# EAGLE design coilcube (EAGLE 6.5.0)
REV: 2v0; TITLE: Coilcube

## Sheet 1 of 2: EPIC & Programmer
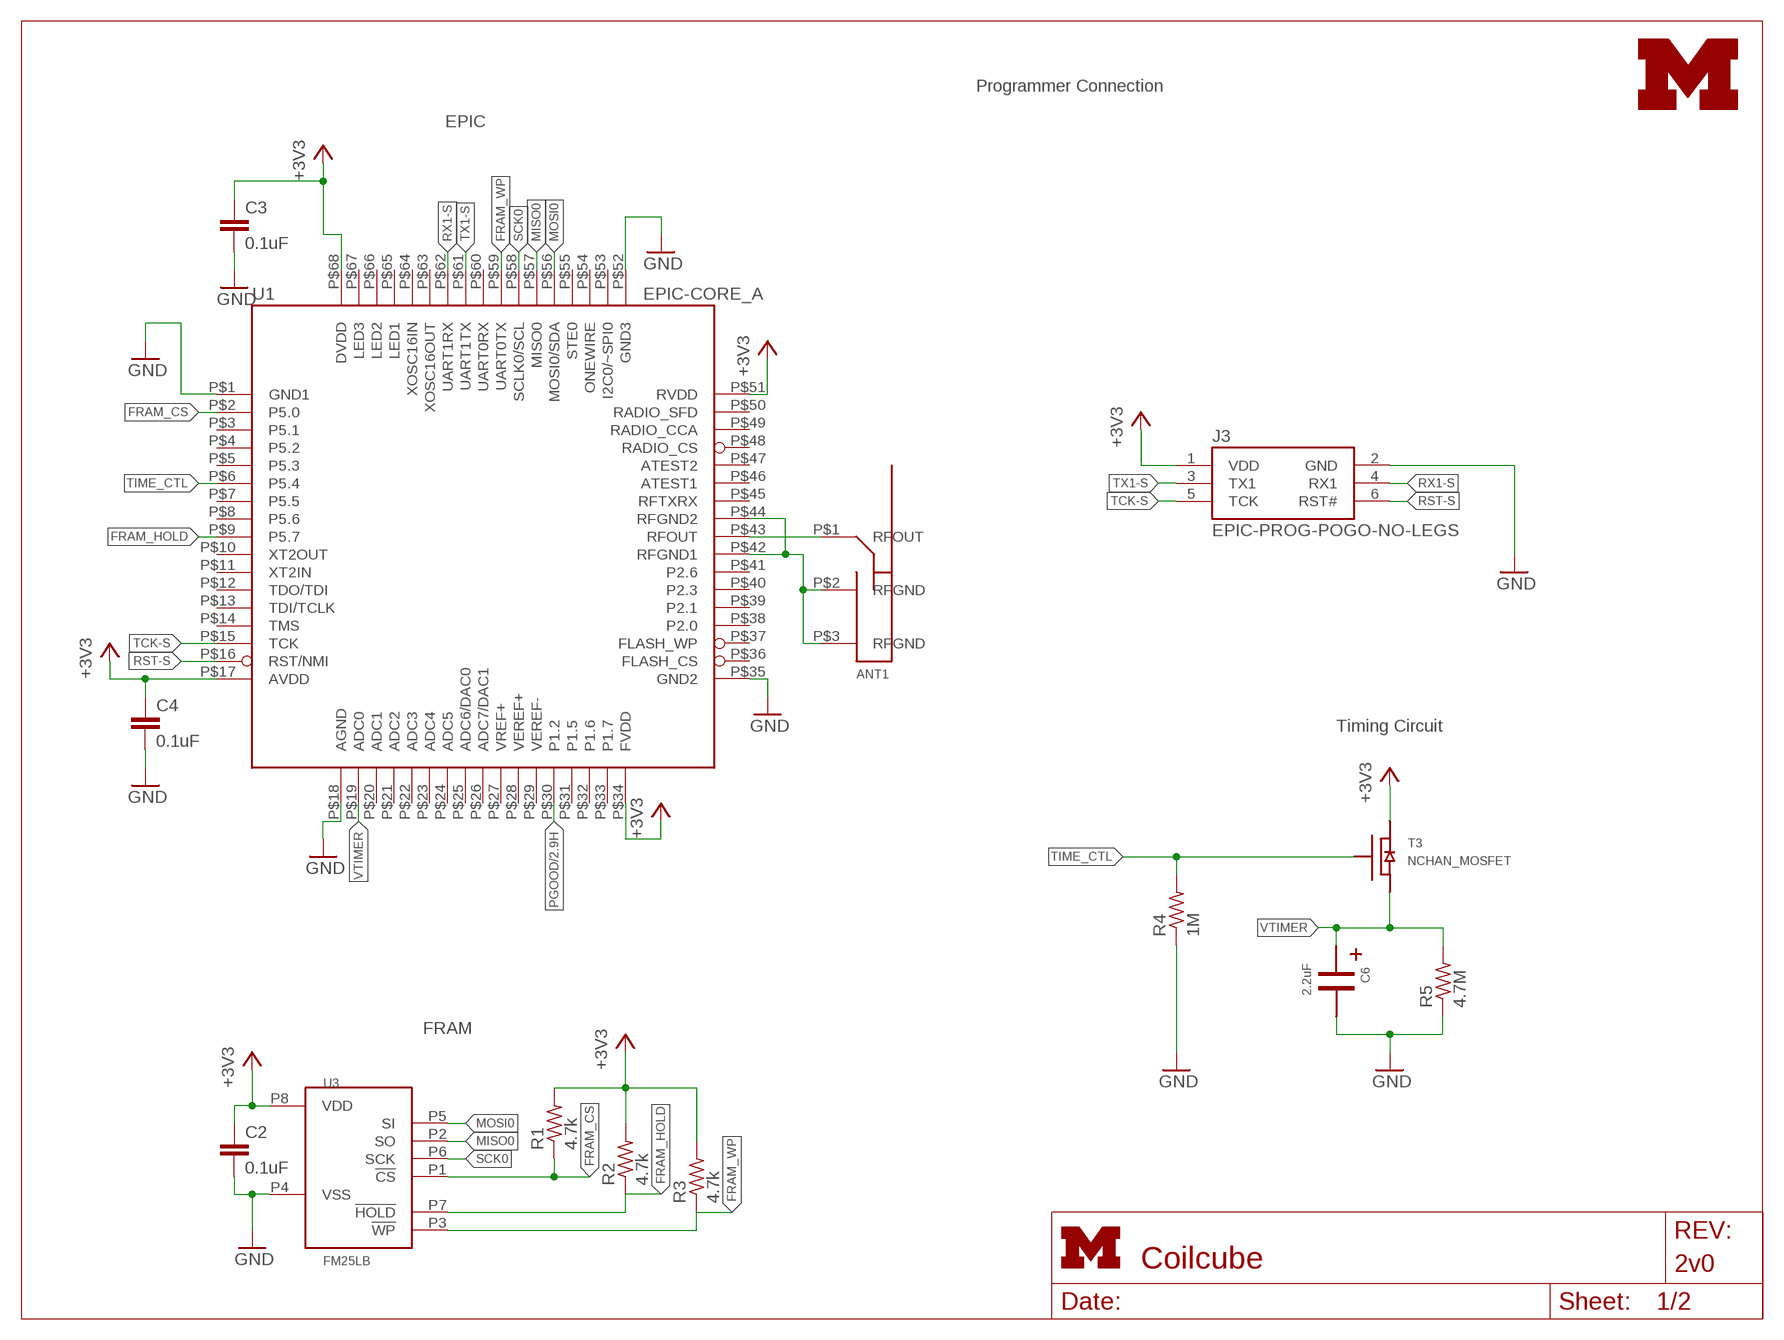
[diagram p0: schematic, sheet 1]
FRAME1 (LETTER_L): HEIGHT: 8.5in; WIDTH: 11in

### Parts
ANT1  PIFA-2.4GHZ  [PIFA-2.4GHZ]
C2  0.1uF  C-EUC0603  [C0603]
C3  0.1uF  C-EUC0603  [C0603]
C4  0.1uF  C-EUC0603  [C0603]
C6  2.2uF  CAP_POLEA1MM5  [CPOL_EEA_1MM5]
J3  EPIC-PROG-POGO-NO-LEGS  [TC2030-IDC-NL]
R1  4.7k  R-US_R0603  [R0603]
R2  4.7k  R-US_R0603  [R0603]
R3  4.7k  R-US_R0603  [R0603]
R4  1M  R-US_R0603  [R0603]
R5  4.7M  R-US_R0603  [R0603]
T3  NCHAN_MOSFET  [NCHAN_MOSFET]
U1  EPIC-CORE_A  [EPIC-LCC68]
U3  FM25LB  [SOIC_8]
U$1  UMICH_SOLID_MEDIUM  [UMICH_SOLID_200MIL]

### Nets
+3V3: C2.1 C3.1 C4.1 J3.1(VDD) R1.2 R2.2 R3.2 T3.D U1.P$17(AVDD) U1.P$34(FVDD) U1.P$51(RVDD) U1.P$68(DVDD) U3.P8(VDD) ; also sheet 2
FRAM_CS: R1.1 U1.P$2(P5.0) U3.P1(!CS)
FRAM_HOLD: R2.1 U1.P$9(P5.7) U3.P7(!HOLD)
FRAM_WP: R3.1 U1.P$59(UART0TX) U3.P3(!WP)
GND: C2.2 C3.2 C4.2 C6.- J3.2(GND) R4.1 R5.1 U1.P$1(GND1) U1.P$18(AGND) U1.P$35(GND2) U1.P$52(GND3) U3.P4(VSS) ; also sheet 2
MISO0: U1.P$57(MISO0) U3.P2(SO)
MOSI0: U1.P$56(MOSI0/SDA) U3.P5(SI)
N$1: ANT1.P$1(RFOUT) U1.P$43(RFOUT)
PGOOD: U1.P$30(P1.2) ; also sheet 2
RFGND: ANT1.P$2(RFGND) ANT1.P$3(RFGND) U1.P$42(RFGND1) U1.P$44(RFGND2)
RST-S: J3.6(RST#) U1.P$16(RST/NMI)
RX1-S: J3.4(RX1) U1.P$62(UART1RX)
SCK0: U1.P$58(SCLK0/SCL) U3.P6(SCK)
TCK-S: J3.5(TCK) U1.P$15(TCK)
TIME_CTL: R4.2 T3.G U1.P$6(P5.4)
TX1-S: J3.3(TX1) U1.P$61(UART1TX)
VTIMER: C6.+ R5.2 T3.S U1.P$19(ADC0)
Unconnected: U1.P$3(P5.1) U1.P$4(P5.2) U1.P$5(P5.3) U1.P$7(P5.5) U1.P$8(P5.6) U1.P$10(XT2OUT) U1.P$11(XT2IN) U1.P$12(TDO/TDI) U1.P$13(TDI/TCLK) U1.P$14(TMS) U1.P$20(ADC1) U1.P$21(ADC2) U1.P$22(ADC3) U1.P$23(ADC4) U1.P$24(ADC5) U1.P$25(ADC6/DAC0) U1.P$26(ADC7/DAC1) U1.P$27(VREF+) U1.P$28(VEREF+) U1.P$29(VEREF-) U1.P$31(P1.5) U1.P$32(P1.6) U1.P$33(P1.7) U1.P$36(FLASH_CS) U1.P$37(FLASH_WP) U1.P$38(P2.0) U1.P$39(P2.1) U1.P$40(P2.3) U1.P$41(P2.6) U1.P$45(RFTXRX) U1.P$46(ATEST1) U1.P$47(ATEST2) U1.P$48(RADIO_CS) U1.P$49(RADIO_CCA) U1.P$50(RADIO_SFD) U1.P$53(I2C0/~SPI0) U1.P$54(ONEWIRE) U1.P$55(STE0) U1.P$60(UART0RX) U1.P$63(XOSC16OUT) U1.P$64(XOSC16IN) U1.P$65(LED1) U1.P$66(LED2) U1.P$67(LED3)

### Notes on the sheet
- Programmer Connection
- EPIC
- Timing Circuit
- FRAM

## Sheet 2 of 2: Power Supply
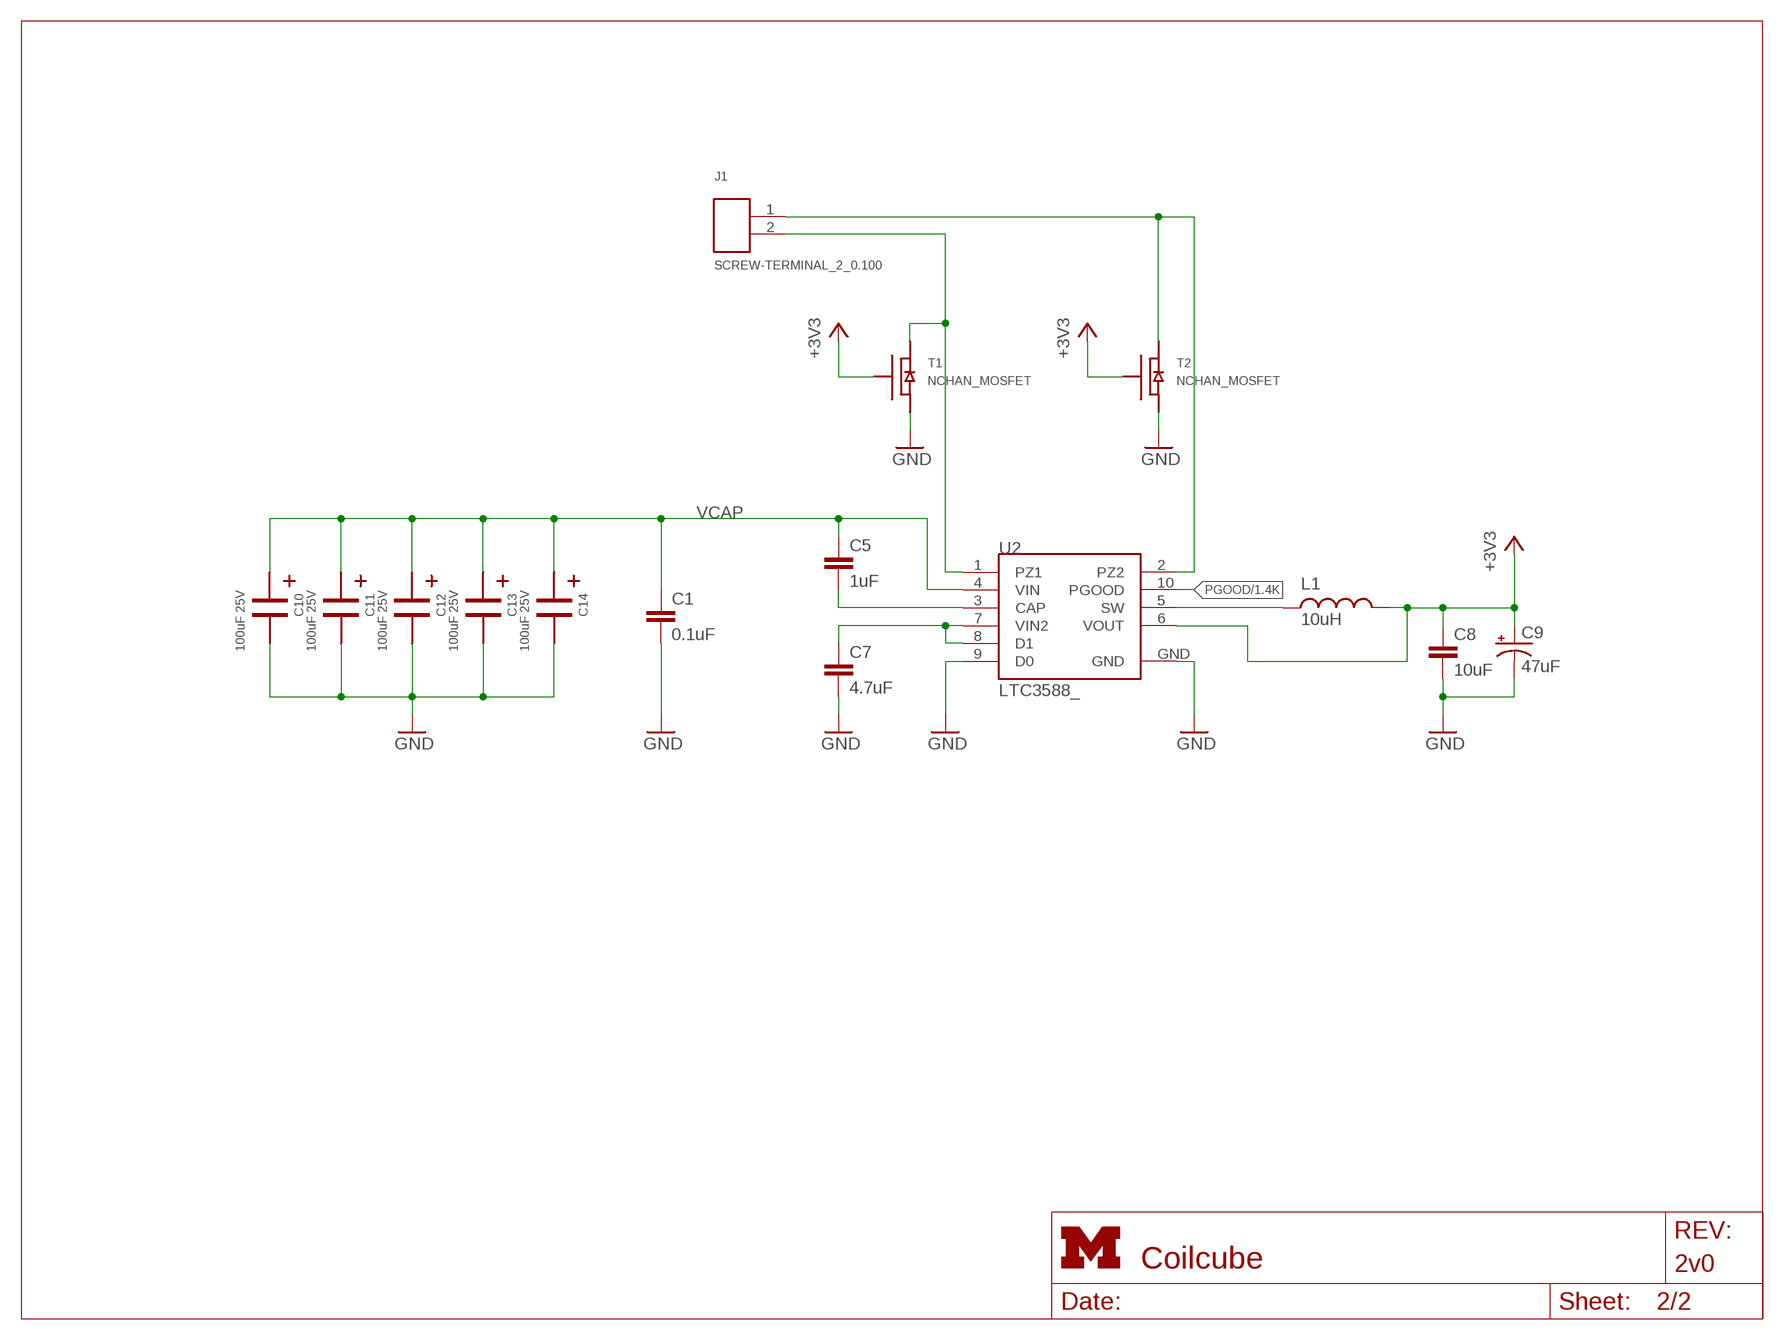
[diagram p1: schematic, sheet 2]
FRAME5 (LETTER_L): HEIGHT: 8.5in; WIDTH: 11in

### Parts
C1  0.1uF  C-EUC0603  [C0603]
C5  1uF  C-EUC0603  [C0603]
C7  4.7uF  C-EUC0603  [C0603]
C8  10uF  C-EUC1206  [C1206]
C9  47uF  CAP_POL1206  [EIA3216]
C10  100uF 25V  2917_CAP_POL  [2917_CAP_POL]
C11  100uF 25V  2917_CAP_POL  [2917_CAP_POL]
C12  100uF 25V  2917_CAP_POL  [2917_CAP_POL]
C13  100uF 25V  2917_CAP_POL  [2917_CAP_POL]
C14  100uF 25V  2917_CAP_POL  [2917_CAP_POL]
J1  SCREW-TERMINAL_2_0.100  [CONN_BLOCK_2]
L1  10uH  INDUCTOR1210  [1210]
T1  NCHAN_MOSFET  [NCHAN_MOSFET]
T2  NCHAN_MOSFET  [NCHAN_MOSFET]
U2  LTC3588_  [MSOP-10-GNDPAD]

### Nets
+3V3: C8.1 C9.A(+) L1.2 T1.G T2.G U2.6(VOUT) ; also sheet 1
GND: C1.2 C7.2 C8.2 C9.C(-) C10.- C11.- C12.- C13.- C14.- T1.S T2.S U2.9(D0) U2.GND ; also sheet 1
N$20: L1.1 U2.5(SW)
N$22: C5.2 U2.3(CAP)
PGOOD: U2.10(PGOOD) ; also sheet 1
PZ1: J1.2 T1.D U2.1(PZ1)
PZ2: J1.1 T2.D U2.2(PZ2)
VCAP: C1.1 C5.1 C10.+ C11.+ C12.+ C13.+ C14.+ U2.4(VIN)
VIN2: C7.1 U2.7(VIN2) U2.8(D1)

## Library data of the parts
ANT1 = berkeley-epic:PIFA-2.4GHZ
C1-C4 = rcl:C-EU: CAPACITOR, European symbol; DIGIKEY: 445-1316-1-ND
C5 = rcl:C-EU: CAPACITOR, European symbol; DIGIKEY: 445-1321-1-ND
C6 = coilcube:CAP_POL; DIGIKEY: P14506-ND
C7 = rcl:C-EU: CAPACITOR, European symbol; DIGIKEY: 445-5178-1-ND
C8 = rcl:C-EU: CAPACITOR, European symbol; DIGIKEY: 399-8152-1-ND
C9 = SparkFun-Passives:CAP_POL: Capacitor Polarized; DIGIKEY: 399-3700-1-ND
C10-C14 = coilcube:2917_CAP_POL; DIGIKEY: 399-5175-1-ND
J1 = headers:SCREW-TERMINAL_2_0.100: 2x 0.100 in screw terminal block; DIGIKEY: 277-1273-ND
J3 = epic:EPIC-PROG-POGO: Epic programmer based on the Tag Connect pogo pin cable.; TAG-CONNECT: TC2030-IDC-NL
L1 = SparkFun-Passives:INDUCTOR: Inductors; DIGIKEY: 587-1625-1-ND
R1-R5 = rcl:R-US_: RESISTOR, American symbol; DIGIKEY: P4.7KGCT-ND
T1 T2 = Power_Metering:NCHAN_MOSFET; DIGIKEY: SI1302DL-T1-GE3CT-ND
T3 = Power_Metering:NCHAN_MOSFET; DIGIKEY: 568-3244-1-ND
U1 = berkeley-epic:EPIC-CORE_A
U2 = SparkFun-PowerIC:LTC3588: Energy Harvesting Power Supply; DIGIKEY: LTC3588EMSE-1#PBF-ND
U3 = coilcube:FM25LB; DIGIKEY: 428-3210-ND
U$1 = logos:UMICH_SOLID

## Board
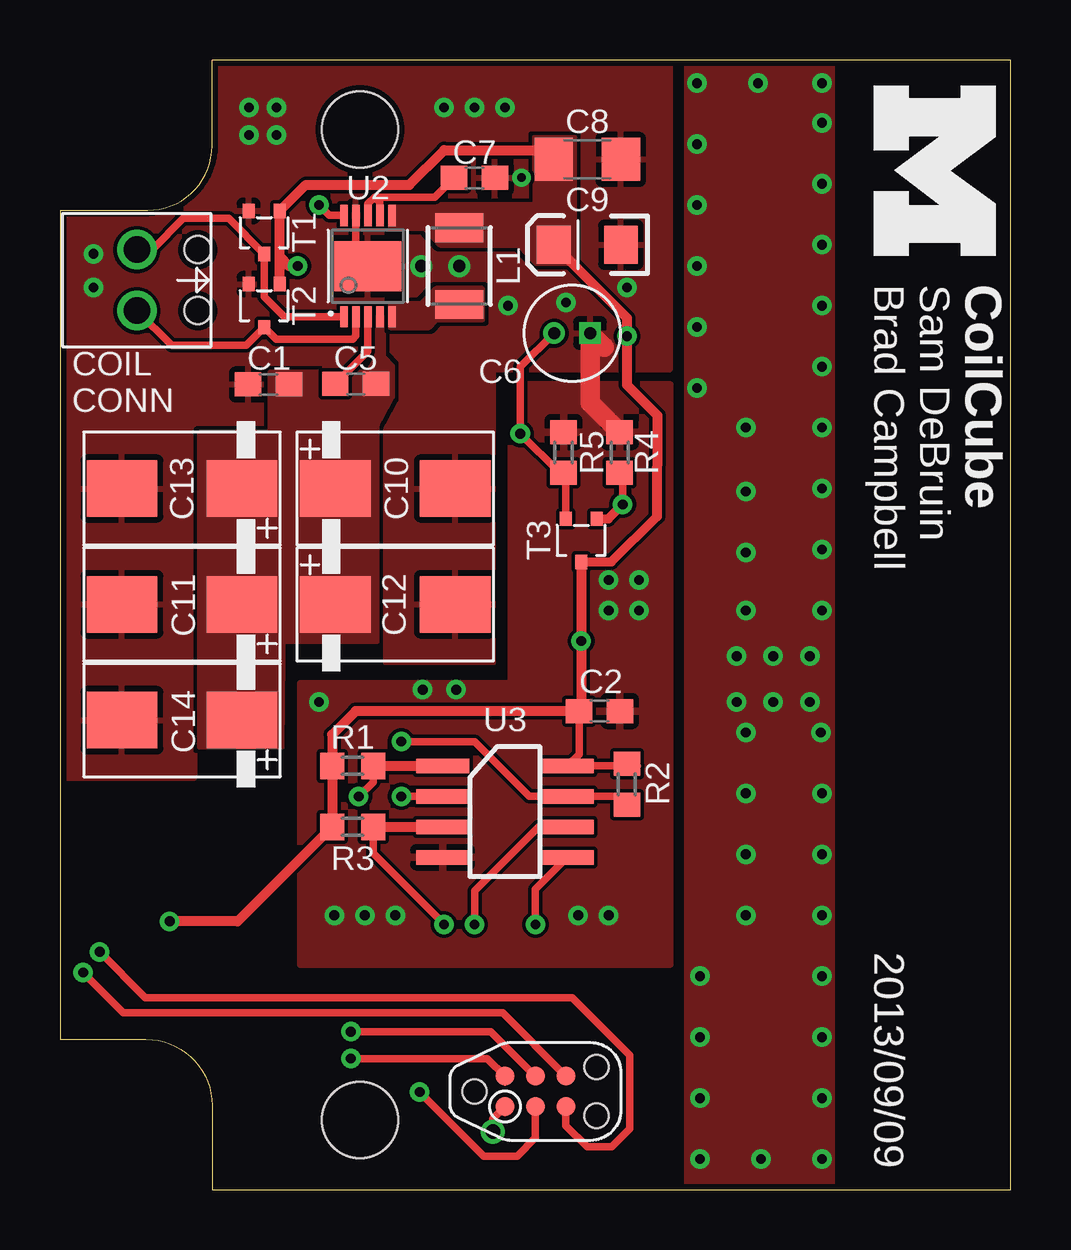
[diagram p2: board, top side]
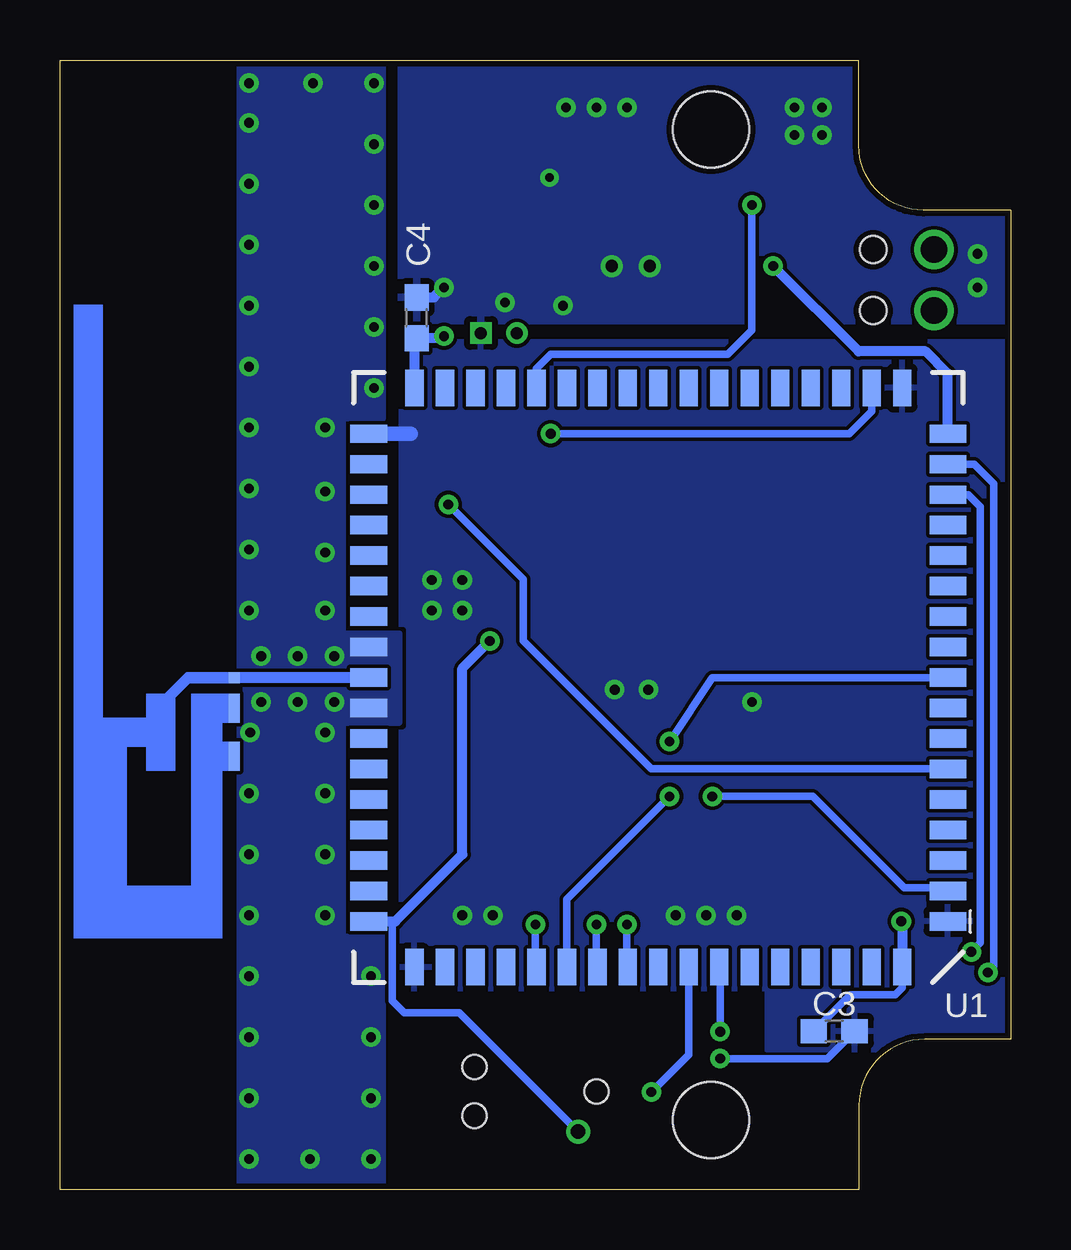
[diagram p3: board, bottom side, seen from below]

Size 39.62 x 47.07 mm. Coordinates in mm from the lower left corner, seen from the top.
Outline: 6.34,0 39.62,0 39.62,47.07 6.34,47.07 6.34,43.49 arc-90 3.65,40.8 0,40.8 0,6.26 3.58,6.26 arc-90 6.34,3.51 6.34,0
Copper layers (1*16): Top 0.0178mm / dielectric 59mil / Bottom 0.0178mm
Design rules "sunstone-2lyr_v1.0.0.3 *": minimum track width 6mil, minimum drill 14mil, track to track 6mil, track to pad 6mil, pad to pad 6mil, via to via 6mil, smd to smd 6mil, copper to edge 10mil, drill to drill 16mil, minimum pad ring 8mil, minimum via ring 8mil, stop-mask expansion 3mil, vias tented up to drill 20mil, thermal gap 10mil
Holes 3.17 mm at 12.5,44.17 12.5,2.9
tKeepout: area 10.1,0.5 to 14.9,5.3; area 10.1,41.8 to 14.9,46.6
Milling: 12 lines

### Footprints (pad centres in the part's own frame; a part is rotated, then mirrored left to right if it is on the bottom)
PIFA-2.4GHZ = smd 0.46 x 0.46: P$1 -2.65,-1.495 | smd 0.46 x 1.2: P$2 -2.655,1.785; P$3 -2.65,-0.215
C0603 = smd 1.1 x 1: 1 -0.85,0; 2 0.85,0
CPOL_EEA_1MM5 = drill 0.5: + 0.75,0 | drill 0.5 square: - -0.75,0
C1206 = smd 1.6 x 1.8: 1 -1.4,0; 2 1.4,0
EIA3216 = smd 1.4 x 1.6: A 1.4,0; C -1.4,0
2917_CAP_POL = smd 2.95 x 2.35: + -2.5,0; - 2.5,0
CONN_BLOCK_2 = drill 1.1: 1 -1.27,0; 2 1.27,0 | hole 1.12: -1.27,-2.54; 1.27,-2.54
TC2030-IDC-NL = smd 0.787 x 0.787: 1 -1.27,-0.635; 2 -1.27,0.635; 3 0,-0.635; 4 0,0.635; 5 1.27,-0.635; 6 1.27,0.635 | hole 1.016: -2.54,0; 2.54,1.016; 2.54,-1.016
1210 = smd 1.2 x 2: 1 -1.6,0; 2 1.6,0
R0603 = smd 1 x 1.1: 1 -0.85,0; 2 0.85,0
NCHAN_MOSFET = smd 0.6 x 0.5: D -0.9,0; G 0.9,-0.65; S 0.9,0.65
EPIC-LCC68 = smd 1.524 x 0.762: P$1 -12.065,10.16; P$2 -12.065,8.89; P$3 -12.065,7.62; P$4 -12.065,6.35; P$5 -12.065,5.08; P$6 -12.065,3.81; P$7 -12.065,2.54; P$8 -12.065,1.27; P$9 -12.065,0; P$10 -12.065,-1.27; P$11 -12.065,-2.54; P$12 -12.065,-3.81; P$13 -12.065,-5.08; P$14 -12.065,-6.35; P$15 -12.065,-7.62; P$16 -12.065,-8.89; P$17 -12.065,-10.16; P$35 12.065,-10.16; P$36 12.065,-8.89; P$37 12.065,-7.62; P$38 12.065,-6.35; P$39 12.065,-5.08; P$40 12.065,-3.81; P$41 12.065,-2.54; P$42 12.065,-1.27; P$43 12.065,0; P$44 12.065,1.27; P$45 12.065,2.54; P$46 12.065,3.81; P$47 12.065,5.08; P$48 12.065,6.35; P$49 12.065,7.62; P$50 12.065,8.89; P$51 12.065,10.16 | smd 0.762 x 1.524: P$18 -10.16,-12.065; P$19 -8.89,-12.065; P$20 -7.62,-12.065; P$21 -6.35,-12.065; P$22 -5.08,-12.065; P$23 -3.81,-12.065; P$24 -2.54,-12.065; P$25 -1.27,-12.065; P$26 0,-12.065; P$27 1.27,-12.065; P$28 2.54,-12.065; P$29 3.81,-12.065; P$30 5.08,-12.065; P$31 6.35,-12.065; P$32 7.62,-12.065; P$33 8.89,-12.065; P$34 10.16,-12.065; P$52 10.16,12.065; P$53 8.89,12.065; P$54 7.62,12.065; P$55 6.35,12.065; P$56 5.08,12.065; P$57 3.81,12.065; P$58 2.54,12.065; P$59 1.27,12.065; P$60 0,12.065; P$61 -1.27,12.065; P$62 -2.54,12.065; P$63 -3.81,12.065; P$64 -5.08,12.065; P$65 -6.35,12.065; P$66 -7.62,12.065; P$67 -8.89,12.065; P$68 -10.16,12.065
MSOP-10-GNDPAD = smd 0.305 x 0.889: 1 -1,-2.11; 2 -0.5,-2.11; 3 0,-2.11; 4 0.5,-2.11; 5 1,-2.11; 6 1,2.11; 7 0.5,2.11; 8 0,2.11; 9 -0.5,2.11; 10 -1,2.11 | smd 2.794 x 2.083: GND 0,0
SOIC_8 = smd 2.2 x 0.6: P1 -2.6,1.905; P2 -2.6,0.635; P3 -2.6,-0.635; P4 -2.6,-1.905; P5 2.6,-1.905; P6 2.6,-0.635; P7 2.6,0.635; P8 2.6,1.905

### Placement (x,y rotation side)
ANT1  35.01,19.84 180 bottom
C1  8.69,33.55 180 top
C2  22.48,19.94 0 top
C3  7.37,6.6 0 bottom
C4  24.77,36.32 90 bottom
C5  12.32,33.58 180 top
C6  21.34,35.69 180 top
C7  17.27,42.15 0 top
C8  21.97,42.93 0 top
C9  21.97,39.37 180 top
C10  13.97,29.21 0 top
C11  5.08,24.38 180 top
C12  13.97,24.38 0 top
C13  5.08,29.21 180 top
C14  5.08,19.56 180 top
J1  3.2,37.9 90 top
J3  19.81,4.09 0 top
L1  16.64,38.48 90 top
R1  12.19,17.65 180 top
R2  23.62,16.89 90 top
R3  12.19,15.11 180 top
R4  23.32,30.71 270 top
R5  20.98,30.71 270 top
T1  8.51,39.88 90 top
T2  8.51,36.83 90 top
T3  21.72,27.05 90 top
U1  14.69,21.34 180 bottom
U2  12.83,38.48 0 top
U3  18.54,15.75 0 top
U$1  33.91,46 270 top

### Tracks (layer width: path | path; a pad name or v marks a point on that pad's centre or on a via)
+3V3  (via drill 0.41, 0.6)
  Top 0.254: 20.32,43.18 C8.1
  Top 0.305: R2.2 23.53,17.65 U3.P8 21.63,18.14 C2.1 | J3.1 18.03,2.95 v18.03,2.41
  Top 0.381: T3.D 22.98,26.15 24.87,28.04
  Top 0.406: T2.G 9.16,38.86 | 9.16,38.86 T1.G 10.24,41.86 14.55,41.86 16,43.31 20.19,43.31 C8.1 | C9.A 23.62,36.32 v23.62,35.56 23.62,33.53 24.89,32.26 24.87,28.04 | T3.D v21.72,22.86 21.72,20.03 C2.1 12.32,19.94 11.34,18.96 R1.2 R3.2 7.41,11.18 v4.57,11.18 | 23.53,17.65 24,17.65 | v9.91,38.48 9.54,38.48 9.16,38.86
  Bottom 0.305: U1.P$68 4.53,8.42 4.83,8.13 6.69,8.13 C3.1 | 25.65,11.18 25.78,11.05 25.78,7.87 25.27,7.37 22.99,7.37 v18.03,2.41
  Bottom 0.406: v23.62,35.56 23.58,35.47 C4.1 24.85,35.38 U1.P$34 | v4.57,11.18 4.53,11.14 U1.P$68 | U1.P$51 25.65,11.18 22.86,13.97 22.86,21.72 v21.72,22.86 | U1.P$17 2.63,34 3.56,34.92 6.35,34.92 v9.91,38.48
  pour Top (no thermals): 15.84,39.37 19.15,39.37 19.84,38.61 21.43,38.61 21.43,43.81 19.78,43.81 19.81,41.02 13.78,41.02 13.78,40.07 15.21,40.07
FRAM_CS  (via drill 0.41)
  Top 0.305: R1.1 13.04,16.98 v12.45,16.38
  Top 0.406: R1.1 U3.P1
  Bottom 0.305: U1.P$2 2.76,12.57 4.45,12.57 8.26,16.38 v12.45,16.38
FRAM_HOLD  (via drill 0.41)
  Top 0.305: R2.1 23.28,16.38 U3.P7 19.56,16.38 17.27,18.67 v14.22,18.67
  Bottom 0.305: U1.P$9 12.45,21.34 v14.22,18.67
FRAM_WP  (via drill 0.41)
  Top 0.305: R3.1 13.04,14.01 v16,11.05
  Top 0.406: R3.1 U3.P3
  Bottom 0.305: v16,11.05 16,9.31 U1.P$59
GND  (via drill 0.36, 0.41, 0.51)
  Top 0.305: U2.9 12.33,38.98 U2.GND | J3.2 17.8,5.46 v12.12,5.46
  Top 0.813: 22.67,35.11 C6.- 22.09,32.79 R4.1
  Bottom 0.305: v12.12,5.46 7.66,5.46 C3.2
  Bottom 0.406: C4.2 24.04,37.17 v23.62,37.59
  Bottom 0.61: U1.P$35 25.02,31.5
  other vias: 15.05,38.48 10.79,20.32 15.11,20.83 16.51,20.83 22.86,25.4 24.13,25.4 24.13,24.13 22.86,24.13 22.86,11.43 21.59,11.43 13.97,11.43 12.7,11.43 11.43,11.43 19.23,42.16 7.87,45.09 9.02,45.09 9.02,43.94 7.87,43.94 21.08,36.96 18.67,36.83 16,45.09 17.27,45.09 18.54,45.09 1.4,38.99 1.4,37.59 16.64,38.48
  pour Bottom (rank 6): 0,35.31 25.4,35.31 25.4,8.38 10.16,8.38 10.16,5.84 0,5.84
  pour Top (rank 6): 0,17.14 0,46.99 25.4,46.99 25.4,34.16 18.03,34.16 18.03,21.97 13.59,21.97 13.59,31.5 5.59,31.5 5.59,17.14
  pour Top: 18.8,33.53 25.4,33.53 25.4,9.4 10.03,9.4 10.03,21.08 18.8,21.08
  pour Bottom: 0,46.99 25.4,46.99 25.4,36.2 0,36.2
MISO0  (via drill 0.41)
  Top 0.305: U3.P2 v14.22,16.38
  Bottom 0.305: v14.22,16.38 18.5,12.1 U1.P$57
MOSI0  (via drill 0.41)
  Top 0.305: U3.P5 19.81,12.51 v19.81,11.05
  Bottom 0.305: v19.81,11.05 19.81,9.31 U1.P$56
N$1
  Bottom 0.406: ANT1.P$1
  Bottom 0.457: U1.P$43 ANT1.P$1
N$20
  pour Top (no thermals): 13.78,36.89 13.78,35.94 15.37,35.94 15.68,36.26 17.59,36.26 17.59,37.53 15.68,37.53 15.05,36.89
N$22
  Top 0.305: C5.2 12.83,34.94 U2.3
PGOOD  (via drill 0.41)
  Top 0.305: U2.10 11.23,40.59 v10.79,41.02
  Bottom 0.305: v10.79,41.02 10.79,35.81 11.81,34.8 19.18,34.8 19.77,34.2 U1.P$30
PZ1
  Top 0.305: U2.1 9.35,36.37 8.51,37.21 T1.D | T1.D | T1.D 7.03,40.46 5.13,40.46 3.83,39.17 J1.2
PZ2
  Top 0.254: 8.52,35.94 T2.D
  Top 0.305: U2.2 12.33,35.57 12.19,35.43 9.01,35.43 T2.D 7.76,35.18 4.65,35.18 J1.1
RFGND  (via drill 0.41)
  other vias: 28.19,22.23 28.19,20.32 28.57,19.05 31.24,22.23 31.24,20.32 31.7,19.05 31.75,16.51 31.75,13.97 31.75,11.43 31.75,8.89 31.75,24.13 31.75,26.67 31.75,31.75 31.75,29.21 31.75,34.29 29.72,22.23 29.72,20.32 28.57,24.13 31.75,36.83 31.75,39.37 31.75,41.91 31.75,44.45 31.75,46.1 26.54,46.1 31.75,6.35 31.75,3.81 31.75,1.27 26.54,43.56 26.54,41.02 26.54,38.48 26.54,35.94 26.54,33.4 28.57,31.75 28.57,29.08 28.57,26.54 28.57,16.51 28.57,13.97 28.57,11.43 26.67,8.89 26.67,6.35 26.67,3.81 26.67,1.27 29.21,1.27 29.08,46.1
  pour Bottom (no thermals): 26.16,47.07 32.16,47.07 32.16,0 26.16,0 26.16,10.54 27.81,10.54 27.81,19.46 25.48,19.46 25.48,23.16 27.81,23.16 27.81,32.13 26.16,32.13
  pour Top: 26.14,47.07 32.16,47.07 32.16,0 26.14,0
RST-S  (via drill 0.41)
  Top 0.305: J3.6 18.44,7.37 2.64,7.37 v0.96,9.04
  Bottom 0.305: U1.P$16 1.52,30.23 0.71,29.41 0.71,9.3 v0.96,9.04
RX1-S  (via drill 0.41)
  Top 0.305: J3.4 17.96,6.58 v12.12,6.58
  Bottom 0.305: v12.12,6.58 12.12,9.23 U1.P$62
SCK0  (via drill 0.41)
  Top 0.305: U3.P6 19.94,15.11 17.27,12.45 v17.27,11.05
  Bottom 0.305: v17.27,11.05 17.27,9.31 U1.P$58
TCK-S  (via drill 0.41)
  Top 0.305: v1.65,9.91 3.56,8 21.34,8 23.75,5.59 23.75,2.54 22.99,1.78 21.97,1.78 21.08,2.67 J3.5
  Bottom 0.305: v1.65,9.91 1.27,10.29 1.27,28.45 1.78,28.96 U1.P$15
TIME_CTL  (via drill 0.41)
  Top 0.305: R4.2 23.44,29.73 v23.44,28.55
  Top 0.381: T3.G 22.85,27.95 v23.44,28.55
  Bottom 0.305: U1.P$6 14.99,17.53 20.32,22.86 20.32,25.43 v23.44,28.55
TX1-S  (via drill 0.41)
  Top 0.305: J3.3 19.81,2.16 19.05,1.4 17.65,1.4 v14.99,4.06
  Bottom 0.305: 13.41,9.26 U1.P$61 13.42,5.63 v14.99,4.06
VCAP
  pour Top (rank 2, no thermals): 13.84,34.29 13.46,34.67 13.46,36.32 13.21,36.32 13.21,34.67 12.83,34.04 8.76,34.04 8.76,31.53 5.83,31.53 5.82,18.45 9.25,18.47 9.27,22.1 9.27,22.86 13.21,22.86 13.21,31.88 13.84,33.05
VIN2
  Top 0.305: U2.8 12.83,41.07 13.11,41.35 | U2.7 13.33,41.13 13.11,41.35 | 13.11,41.35 15.62,41.35 C7.1
VTIMER  (via drill 0.41)
  Top 0.305: T3.S 21.07,29.77 R5.2 20.81,29.86 v19.18,31.5 19.18,34.28 C6.+
  Bottom 0.305: v19.18,31.5 6.73,31.5 5.8,32.42 U1.P$19

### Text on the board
tPlace: Brad Campbell | Sam DeBruin | CoilCube | COIL / CONN | 2013/09/09

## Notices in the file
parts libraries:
SparkFun-PowerIC: Licensing: CC v3.0 Share-Alike You are welcome to use this library for commercial purposes.
